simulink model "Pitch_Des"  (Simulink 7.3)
settings: Solver=ode45  StartTime=0.0  StopTime=100  RelTol=1e-3
undefined symbols (not defined in the file or in its folder): Ap, Bp, Cp, Dp

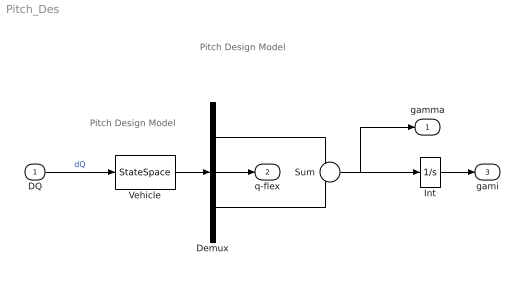
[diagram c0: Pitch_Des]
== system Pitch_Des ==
  note: Pitch Design Model
  note: Pitch Design Model
  DQ : Inport  OutDataType=sfix(16)  OutScaling=2^0
  Demux : Demux  Outputs=3
  Int : Integrator
  Sum : Sum  Inputs=+-  OutDataType=sfix(16)  OutScaling=2^0
  Vehicle : StateSpace  A=Ap  B=Bp  C=Cp  D=Dp
  gamma : Outport  OutDataType=sfix(16)  OutScaling=2^0
  q-flex : Outport  Port=2  OutDataType=sfix(16)  OutScaling=2^0
  gami : Outport  Port=3  OutDataType=sfix(16)  OutScaling=2^0
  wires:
  Vehicle/1 -> Demux/1
  Sum/1 -> Int/1, gamma/1
  Demux/1 -> Sum/1
  Demux/2 -> q-flex/1
  Demux/3 -> Sum/2
  DQ/1 -> Vehicle/1  "dQ"
  Int/1 -> gami/1
